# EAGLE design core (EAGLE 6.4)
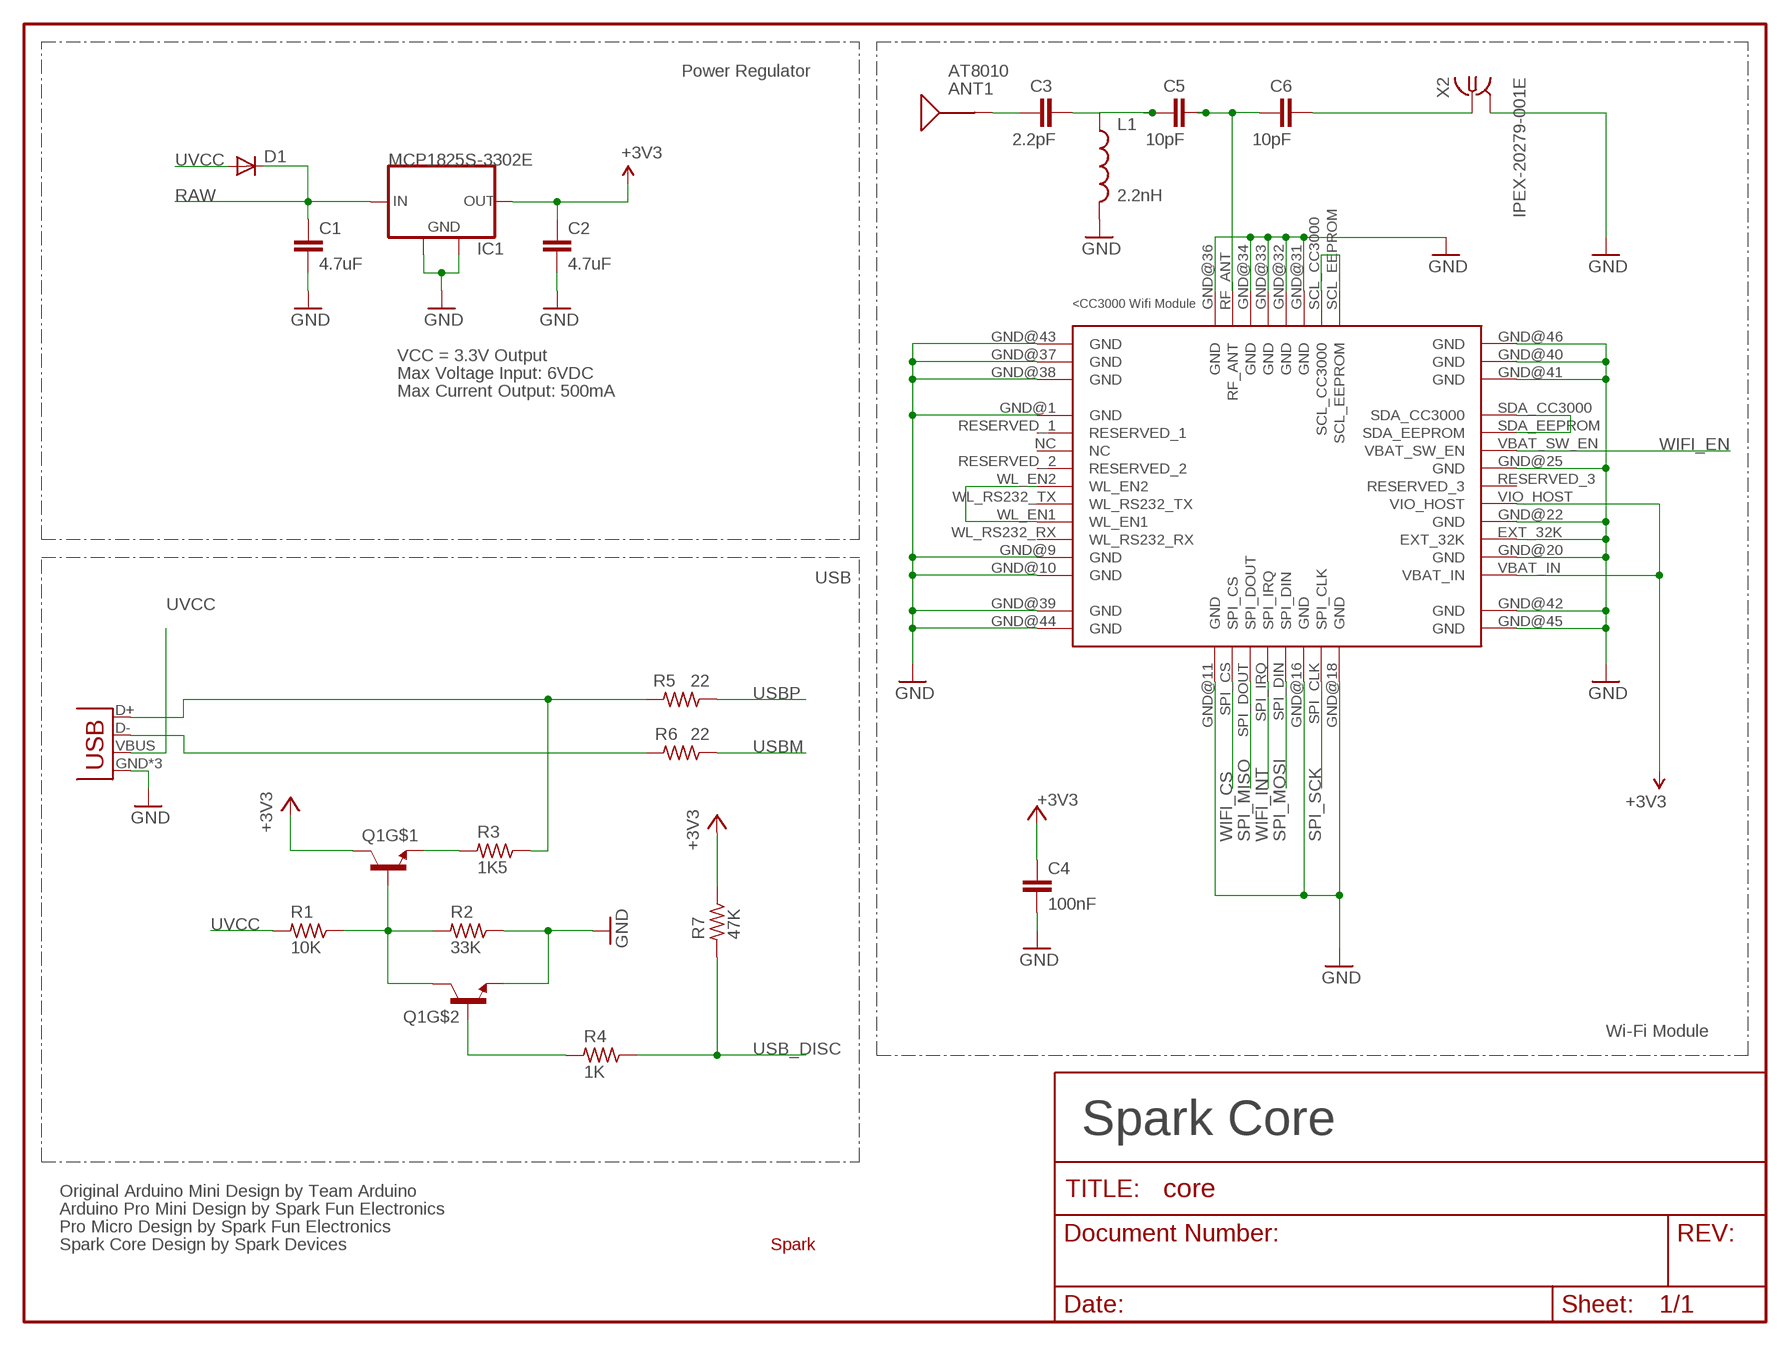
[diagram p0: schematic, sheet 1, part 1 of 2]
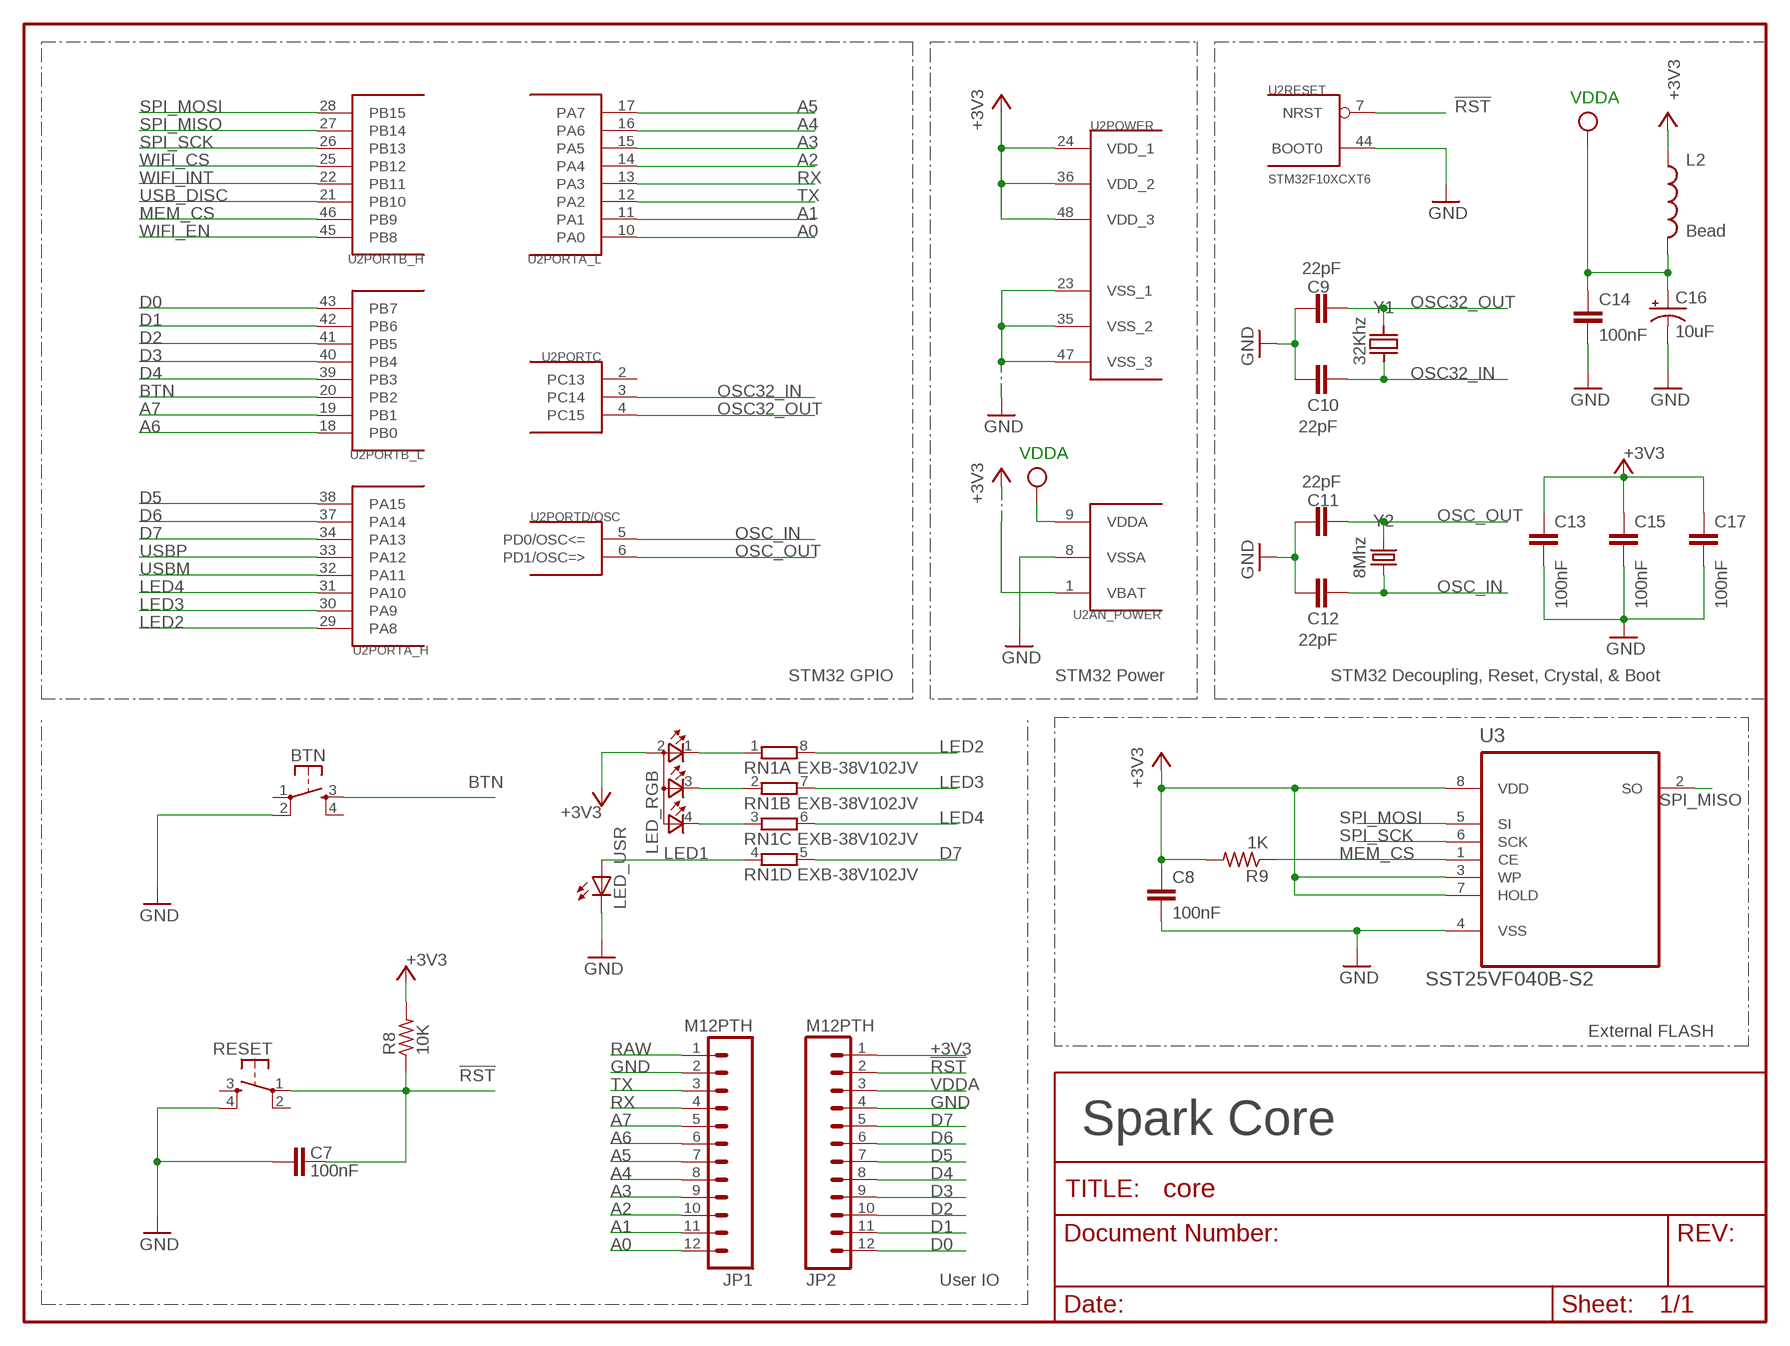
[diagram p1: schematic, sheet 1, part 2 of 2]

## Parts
ANT1  AT8010  [AT8010]
BTN  KMR211GLFS  TAC_SWITCHSMD  [TACTILE_SWITCH_SMD]
C1  4.7uF  C-EUC0603  [C0603]
C2  4.7uF  C-EUC0603  [C0603]
C3  2.2pF  C-EUC0603  [C0603]
C4  100nF  C-EUC0603  [C0603]
C5  10pF  C-EUC0603  [C0603]
C6  10pF  C-EUC0603  [C0603]
C7  100nF  C-EUC0603  [C0603]
C8  100nF  C-EUC0603  [C0603]
C9  22pF  C-EUC0603  [C0603]
C10  22pF  C-EUC0603  [C0603]
C11  22pF  C-EUC0603  [C0603]
C12  22pF  C-EUC0603  [C0603]
C13  100nF  C-EUC0603  [C0603]
C14  100nF  C-EUC0603  [C0603]
C15  100nF  C-EUC0603  [C0603]
C16  10uF  TANT-CAP1206  [EIA3216]
C17  100nF  C-EUC0603  [C0603]
D1  DIODESOD  [SOD-323]
IC1  MCP1825S-3302E  MCP1825S-SOT223  [SOT223]
JP1  M12PTH  [1X12-SMALL-PADS]
JP2  M12PTH  [1X12-SMALL-PADS]
L1  2.2nH  INDUCTOR0603  [0603]
L2  Bead  INDUCTOR0603  [0603]
LED_RGB  TOPLED-3PLCC  [P-LCC-4-3]
LED_USR  LED0603  [LED-0603]
Q1  MMDT3904  [SOT363]
R1  10K  R-US_R0603  [R0603]
R2  33K  R-US_R0603  [R0603]
R3  1K5  R-US_R0603  [R0603]
R4  1K  R-US_R0603  [R0603]
R5  22  R-US_R0603  [R0603]
R6  22  R-US_R0603  [R0603]
R7  47K  R-US_R0603  [R0603]
R8  10K  R-US_R0603  [R0603]
R9  1K  R-US_R0603  [R0603]
RESET  KMR211GLFS  TAC_SWITCHSMD  [TACTILE_SWITCH_SMD]
RN1  EXB-38V102JV  4R-NEXB38V  [EXB38V]
U1  CC3000  [CC3000]
U2  STM32F10XCXT6  [TQFP48]
U3  SST25VF040B-S2  [SOIC127P790X216-8N]
U$1  SPARK_LOGO2  [SPARK_LOGO2]
X1  USB-MICROB  USBUSB-MICROB-SLOT-HOLE  [USB-MICROB-SLOT-HOLE]
X2  IPEX-20279-001E  [IPEX-20279-001E]
Y1  32Khz  Q_FC135  [FC135]
Y2  8Mhz  CRYSTAL5X3  [CRYSTAL-SMD-5X3]

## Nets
!RST: C7.2 JP2.2 R8.1 RESET.1 U2.7(RESET:NRST)
+3V3: C2.1 C4.1 C8.1 C13.1 C15.1 C17.1 IC1.3(OUT) JP2.1 L2.1 LED_RGB.2(A2) Q1.3(C) R7.1 R8.2 R9.2 U1.VBAT_IN U1.VIO_HOST U2.1(AN_POWER:VBAT) U2.24(POWER:VDD_1) U2.36(POWER:VDD_2) U2.48(POWER:VDD_3) U3.3(WP) U3.7(HOLD) U3.8(VDD)
A0: JP1.12 U2.10(PORTA_L:PA0)
A1: JP1.11 U2.11(PORTA_L:PA1)
A2: JP1.10 U2.14(PORTA_L:PA4)
A3: JP1.9 U2.15(PORTA_L:PA5)
A4: JP1.8 U2.16(PORTA_L:PA6)
A5: JP1.7 U2.17(PORTA_L:PA7)
A6: JP1.6 U2.18(PORTB_L:PB0)
A7: JP1.5 U2.19(PORTB_L:PB1)
BTN: BTN.3 U2.20(PORTB_L:PB2)
D0: JP2.12 U2.43(PORTB_L:PB7)
D1: JP2.11 U2.42(PORTB_L:PB6)
D2: JP2.10 U2.41(PORTB_L:PB5)
D3: JP2.9 U2.40(PORTB_L:PB4)
D4: JP2.8 U2.39(PORTB_L:PB3)
D5: JP2.7 U2.38(PORTA_H:PA15)
D6: JP2.6 U2.37(PORTA_H:PA14)
D7: JP2.5 RN1.5 U2.34(PORTA_H:PA13)
GND [vcc]: BTN.2 C1.2 C2.2 C4.2 C7.1 C8.2 C9.2 C10.2 C11.2 C12.2 C13.2 C14.2 C15.2 C16.C(-) C17.2 IC1.2(GND) IC1.4(GND) JP1.2 JP2.4 L1.2 LED_USR.C Q1.1(E) R2.1 RESET.4 U1.EXT_32K U1.GND@1(GND) U1.GND@9(GND) U1.GND@10(GND) U1.GND@11(GND) U1.GND@16(GND) U1.GND@18(GND) U1.GND@20(GND) U1.GND@22(GND) U1.GND@25(GND) U1.GND@31(GND) U1.GND@32(GND) U1.GND@33(GND) U1.GND@34(GND) U1.GND@36(GND) U1.GND@37(GND) U1.GND@38(GND) U1.GND@39(GND) U1.GND@40(GND) U1.GND@41(GND) U1.GND@42(GND) U1.GND@43(GND) U1.GND@44(GND) U1.GND@45(GND) U1.GND@46(GND) U2.8(AN_POWER:VSSA) U2.23(POWER:VSS_1) U2.35(POWER:VSS_2) U2.44(RESET:BOOT0) U2.47(POWER:VSS_3) U3.4(VSS) X1.GND X1.MT1(GND) X1.MT2(GND) X2.2@1(GND) X2.2@2(GND)
LED1: LED_USR.A RN1.4
LED2: RN1.8 U2.29(PORTA_H:PA8)
LED3: RN1.7 U2.30(PORTA_H:PA9)
LED4: RN1.6 U2.31(PORTA_H:PA10)
MEM_CS: R9.1 U2.46(PORTB_H:PB9) U3.1(CE)
N$1: R3.1 R5.2 X1.D+
N$2 [RF]: C6.2 X2.1
N$3 [RF]: ANT1.SIG(SIGNAL) C3.1
N$4 [RF]: C5.2 C6.1 U1.RF_ANT
N$5 [RF]: C3.2 C5.1 L1.1
N$6: R6.2 X1.D-
N$7: U1.SCL_CC3000 U1.SCL_EEPROM
N$8: Q1.2(B) R4.2
N$9: U1.WL_EN1 U1.WL_EN2
N$10: LED_RGB.1(CRED) RN1.1
N$12: LED_RGB.3(CBLUE) RN1.2
N$13: Q1.5(B) Q1.6(C) R1.1 R2.2
N$14: LED_RGB.4(CGREEN) RN1.3
N$15: U1.SDA_CC3000 U1.SDA_EEPROM
N$16: Q1.4(E) R3.2
OSC32_IN: C10.1 U2.3(PORTC:PC14) Y1.X1
OSC32_OUT: C9.1 U2.4(PORTC:PC15) Y1.X2
OSC_IN: C12.1 U2.5(PORTD/OSC:PD0/OSC<=) Y2.1
OSC_OUT: C11.1 U2.6(PORTD/OSC:PD1/OSC=>) Y2.3
RAW [vcc]: C1.1 D1.1(C) IC1.1(IN) JP1.1
RX: JP1.4 U2.13(PORTA_L:PA3)
SPI_MISO: U1.SPI_DOUT U2.27(PORTB_H:PB14) U3.2(SO)
SPI_MOSI: U1.SPI_DIN U2.28(PORTB_H:PB15) U3.5(SI)
SPI_SCK: U1.SPI_CLK U2.26(PORTB_H:PB13) U3.6(SCK)
TX: JP1.3 U2.12(PORTA_L:PA2)
USB_DISC: R4.1 R7.2 U2.21(PORTB_H:PB10)
USBM: R6.1 U2.32(PORTA_H:PA11)
USBP: R5.1 U2.33(PORTA_H:PA12)
UVCC: D1.2(A) R1.2 X1.VBUS
VDDA: C14.1 C16.A(+) JP2.3 L2.2 U2.9(AN_POWER:VDDA) ; supply symbol labelled VCC
WIFI_CS: U1.SPI_CS U2.25(PORTB_H:PB12)
WIFI_EN: U1.VBAT_SW_EN U2.45(PORTB_H:PB8)
WIFI_INT: U1.SPI_IRQ U2.22(PORTB_H:PB11)
Unconnected: BTN.1 BTN.4 RESET.2 RESET.3 U1.NC U1.RESERVED_1 U1.RESERVED_2 U1.RESERVED_3 U1.WL_RS232_RX U1.WL_RS232_TX U2.2(PORTC:PC13)

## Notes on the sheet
- Power Regulator
- VDDA
- VCC = 3.3V Output
- Max Voltage Input: 6VDC
- Max Current Output: 500mA
- VDDA
- USB
- STM32 GPIO | STM32 Power | STM32 Decoupling, Reset, Crystal, & Boot
- Wi-Fi Module | External FLASH
- Spark Core | Spark Core
- Original Arduino Mini Design by Team Arduino
- Arduino Pro Mini Design by Spark Fun Electronics
- Pro Micro Design by Spark Fun Electronics
- Spark Core Design by Spark Devices
- User IO

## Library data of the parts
ANT1 = Spark:AT8010: AT8010 Series Multilayer Chip Antenna
BTN RESET = Spark:TAC_SWITCH: SMD Tactiile Switch
C1-C15 C17 = rcl:C-EU: CAPACITOR, European symbol
C16 = Spark:TANT-CAP: Tantalum SMT
D1 = SparkFun:DIODE: Diode
IC1 = Spark:MCP1825S: 500 mA, Low Voltage, Low Quiescent Current LDO Regulator
JP1 JP2 = Spark:M12: Header 12 Standard 12-pin 0.1" header. Use with straight break away headers (SKU : PRT-00116), right angle break away headers (PRT-00553), swiss pins (PRT-00743), machine pins (PRT-00117), and female headers (PRT-00115).
L1 L2 = SparkFun-Passives:INDUCTOR: Inductors
LED_RGB = Spark:TOPLED-3: Cree CLVBA-FKA
LED_USR = SparkFun:LED: LEDs
Q1 = SparkFun-DiscreteSemi:MMDT3904: Dual NPN transistor
R1-R9 = rcl:R-US_: RESISTOR, American symbol
RN1 = resistor-dil:4R-N: Array Chip Resistor Source: RS Component / Phycomp; OC_FARNELL: unknown; OC_NEWARK: unknown
U1 = CC3000:CC3000
U2 = stm32:STM32F10XCXT6: ST STM32F101/103 48pin LQFP
U3 = Spark:SST25VF040B: 4 Mbit SPI Serial Flash
U$1 = Spark:SPARK_LOGO2
X1 = Spark:USB
X2 = Spark:IPEX-20279-001E: Ultra Miniature Coaxial SMT RF Receptacle
Y1 = Spark:Q
Y2 = SparkFun-FreqCtrl:CRYSTAL: Various standard crystals. Proven footprints. Spark Fun Electronics SKU : COM-00534

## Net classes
2 RF: width 0.635 mm, clearance 0.762 mm

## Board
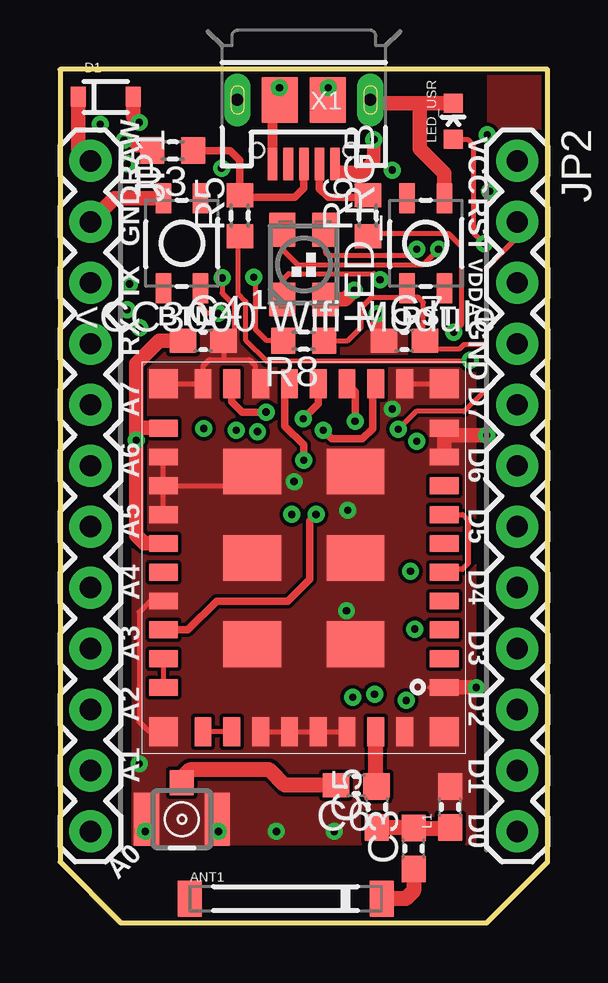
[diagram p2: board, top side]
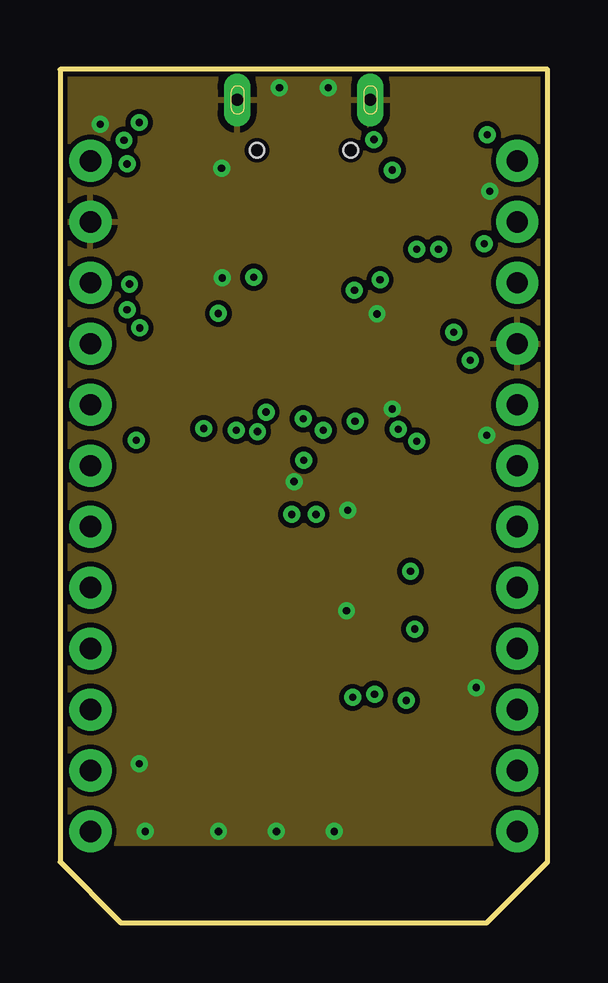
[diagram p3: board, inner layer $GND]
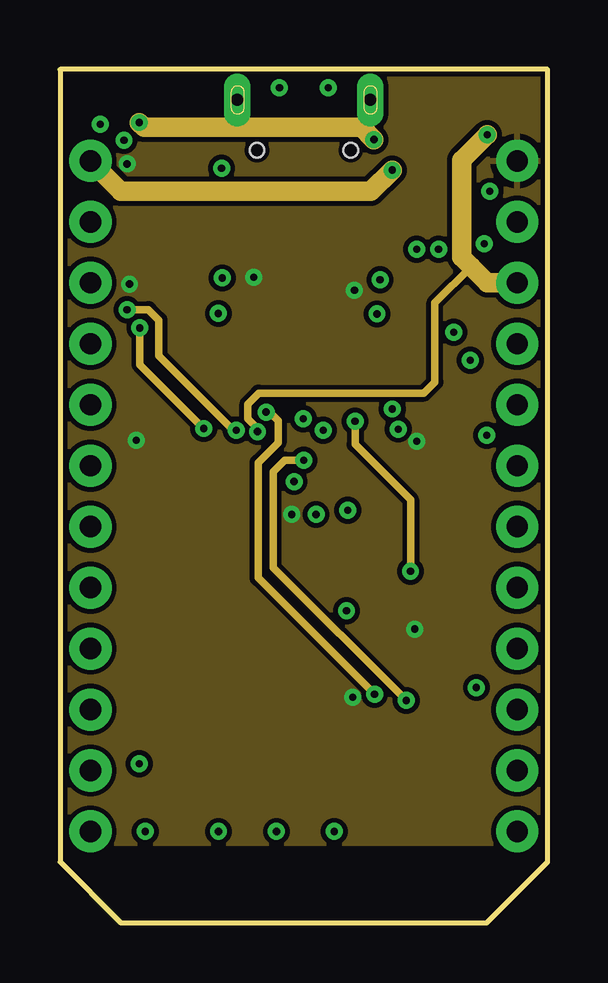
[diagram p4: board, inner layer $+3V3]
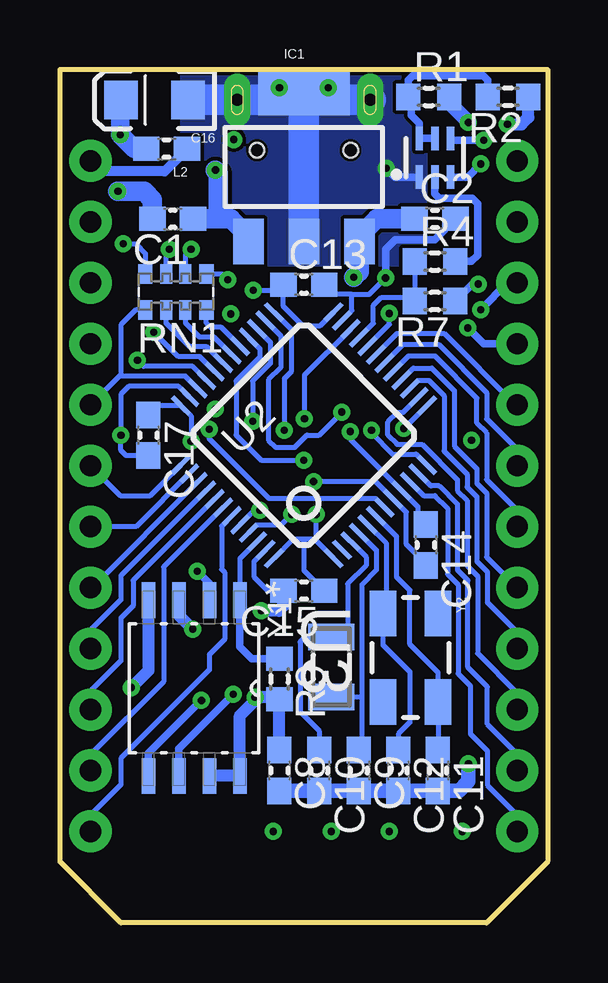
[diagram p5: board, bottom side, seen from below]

Size 20.32 x 35.56 mm. Coordinates in mm from the lower left corner, seen from the top.
Outline: 0,35.56 0,2.54 2.54,0 17.78,0 20.32,2.54 20.32,35.56 0,35.56
Copper layers (1+2*15+16): Top 0.035mm / dielectric 1.5mm / $GND 0.035mm / dielectric 0.15mm / $+3V3 0.035mm / dielectric 0.2mm / Bottom 0.035mm
Design rules "spark": minimum track width 6mil, minimum drill 0.3mm, track to track 6mil, track to pad 6mil, pad to pad 6mil, via to via 6mil, smd to smd 6mil, copper to edge 6mil, drill to drill 6mil, minimum pad ring 12mil, minimum via ring 8mil, stop-mask expansion 4mil, vias tented up to drill 20mil, thermal gap 10mil

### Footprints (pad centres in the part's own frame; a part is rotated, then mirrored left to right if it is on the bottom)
AT8010 = smd 1 x 1.5: NC -4,0; SIG 4,0
TACTILE_SWITCH_SMD = smd 1.25 x 0.65: 1 -1.875,0.775; 2 1.875,0.775; 3 -1.875,-0.775; 4 1.875,-0.775
C0603 = smd 1.1 x 1: 1 -0.85,0; 2 0.85,0
EIA3216 = smd 1.4 x 1.6: A 1.4,0; C -1.4,0
SOD-323 = smd 0.63 x 0.83: 1 -1.15,0; 2 1.15,0
SOT223 = smd 1.27 x 1.905: 1 -2.311,-3.099; 2 0,-3.099; 3 2.311,-3.099 | smd 3.81 x 1.905: 4 0,3.099
1X12-SMALL-PADS = drill 0.889 pad 1.753: 1 0,0; 2 2.54,0; 3 5.08,0; 4 7.62,0; 5 10.16,0; 6 12.7,0; 7 15.24,0; 8 17.78,0; 9 20.32,0; 10 22.86,0; 11 25.4,0; 12 27.94,0
0603 = smd 1.1 x 1: 1 -0.85,0; 2 0.85,0
P-LCC-4-3 = smd 1.1 x 1.4: 1 -0.9,-1.45; 2 0.9,-1.45; 3 0.9,1.45; 4 -0.9,1.45
LED-0603 = smd 0.8 x 0.8: A 0,-0.75; C 0,0.75
SOT363 = smd 0.3 x 0.99: 1 -0.65,-0.8; 2 0,-0.8; 3 0.65,-0.8; 4 0.65,0.81; 5 0,0.81; 6 -0.65,0.81
R0603 = smd 1 x 1.1: 1 -0.85,0; 2 0.85,0
EXB38V = smd 0.6 x 0.8: 1 -1.275,-0.75; 4 1.275,-0.75; 5 1.275,0.75; 8 -1.275,0.75 | smd 0.5 x 0.8: 2 -0.4,-0.75; 3 0.4,-0.75; 6 0.4,0.75; 7 -0.4,0.75
CC3000 = smd 1.2 x 0.7: EXT_32K 5.85,-2.97; GND@1 -5.85,5.43; GND@9 -5.85,-4.17; GND@10 -5.85,-5.37; GND@20 5.85,-4.17; GND@22 5.85,-1.77; GND@25 5.85,1.83; NC -5.85,3.03; RESERVED_1 -5.85,4.23; RESERVED_2 -5.85,1.83; RESERVED_3 5.85,0.63; SDA_CC3000 5.85,5.43; SDA_EEPROM 5.85,4.23; VBAT_IN 5.85,-5.37; VBAT_SW_EN 5.85,3.03; VIO_HOST 5.85,-0.57; WL_EN1 -5.85,-1.77; WL_EN2 -5.85,0.63; WL_RS232_RX -5.85,-2.97; WL_RS232_TX -5.85,-0.57 | smd 0.7 x 1.2: GND@11 -4.2,-7.22; GND@16 1.8,-7.22; GND@18 4.2,-7.22; GND@31 1.8,7.28; GND@32 0.6,7.28; GND@33 -0.6,7.28; GND@34 -1.8,7.28; GND@36 -4.2,7.28; RF_ANT -3,7.28; SCL_CC3000 3,7.28; SCL_EEPROM 4.2,7.28; SPI_CLK 3,-7.22; SPI_CS -3,-7.22; SPI_DIN 0.6,-7.22; SPI_DOUT -1.8,-7.22; SPI_IRQ -0.6,-7.22 | smd 2.4 x 1.9: GND@37 -2.15,3.63; GND@38 -2.15,0.03; GND@39 -2.15,-3.57; GND@40 2.15,3.63; GND@41 2.15,0.03; GND@42 2.15,-3.57 | smd 1.2 x 1.2: GND@43 -5.85,7.28; GND@44 -5.85,-7.22; GND@45 5.85,-7.22; GND@46 5.85,7.28
TQFP48 = smd 0.2 x 1: 1 -2.75,-4.5; 2 -2.25,-4.5; 3 -1.75,-4.5; 4 -1.25,-4.5; 5 -0.75,-4.5; 6 -0.25,-4.5; 7 0.25,-4.5; 8 0.75,-4.5; 9 1.25,-4.5; 10 1.75,-4.5; 11 2.25,-4.5; 12 2.75,-4.5; 25 2.75,4.5; 26 2.25,4.5; 27 1.75,4.5; 28 1.25,4.5; 29 0.75,4.5; 30 0.25,4.5; 31 -0.25,4.5; 32 -0.75,4.5; 33 -1.25,4.5; 34 -1.75,4.5; 35 -2.25,4.5; 36 -2.75,4.5 | smd 1 x 0.2: 13 4.5,-2.75; 14 4.5,-2.25; 15 4.5,-1.75; 16 4.5,-1.25; 17 4.5,-0.75; 18 4.5,-0.25; 19 4.5,0.25; 20 4.5,0.75; 21 4.5,1.25; 22 4.5,1.75; 23 4.5,2.25; 24 4.5,2.75; 37 -4.5,2.75; 38 -4.5,2.25; 39 -4.5,1.75; 40 -4.5,1.25; 41 -4.5,0.75; 42 -4.5,0.25; 43 -4.5,-0.25; 44 -4.5,-0.75; 45 -4.5,-1.25; 46 -4.5,-1.75; 47 -4.5,-2.25; 48 -4.5,-2.75
SOIC127P790X216-8N = smd 1.499 x 0.559: 1 -3.658,1.905; 2 -3.658,0.635; 3 -3.658,-0.635; 4 -3.658,-1.905; 5 3.658,-1.905; 6 3.658,-0.635; 7 3.658,0.635; 8 3.658,1.905
USB-MICROB-SLOT-HOLE = smd 0.4 x 1.35: D+ 0,2.675; D- -0.65,2.675; GND 1.3,2.675; ID 0.65,2.675; VBUS -1.3,2.675 | drill 0.5 pad 1.1 long: MT1 -2.775,0; MT2 2.775,0 | smd 1.5 x 1.9: P$1 -1,0; P$2 1,0.01 | hole 0.6: -1.95,2.1; 1.95,2.1
IPEX-20279-001E = smd 1 x 1.05: 1 0,1.528 | smd 1.05 x 2.2: 2@1 -1.475,0; 2@2 1.475,0
FC135 = smd 1.1 x 1.9: X1 -1.25,0; X2 1.25,0
CRYSTAL-SMD-5X3 = smd 1.9 x 1.1: 1 -1.85,-1.15; 2 1.85,-1.15; 3 1.85,1.15; 4 -1.85,1.15

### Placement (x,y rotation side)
ANT1  9.4,1.02 0 top
BTN  5.08,28.32 90 top
C1  15.62,29.34 180 bottom
C2  4.7,29.34 0 bottom
C3  14.73,3.1 90 top
C4  5.97,24.26 0 top
C5  13.21,4.83 90 top
C6  12.34,5.74 180 top
C7  14.35,24.26 0 top
C8  11.18,6.35 270 bottom
C9  7.87,6.35 270 bottom
C10  9.53,6.35 270 bottom
C11  4.57,6.35 270 bottom
C12  6.22,6.35 270 bottom
C13  10.16,26.59 0 bottom
C14  5.08,15.75 270 bottom
C15  10.16,13.84 180 bottom
C16  16.38,34.29 180 bottom
C17  16.64,20.32 270 bottom
D1  1.91,34.42 0 top
IC1  10.16,31.5 0 bottom
JP1  1.27,31.75 270 top
JP2  19.05,31.75 270 top
L1  16.26,4.83 90 top
L2  15.88,32.26 180 bottom
LED_RGB  10.16,27.43 0 top
LED_USR  16.38,33.4 0 top
Q1  4.7,31.88 0 bottom
R1  4.95,34.42 0 bottom
R2  1.65,34.42 180 bottom
R3  4.7,32.18 180 top
R4  4.7,27.56 0 bottom
R5  7.49,29.46 90 top
R6  12.83,29.46 90 top
R7  4.7,25.91 180 bottom
R8  10.16,24.26 180 top
R9  11.18,10.16 270 bottom
RESET  15.24,28.32 90 top
RN1  15.49,26.29 180 bottom
U1  10.16,15.24 180 top
U2  10.16,20.32 45 bottom
U3  14.73,9.78 270 bottom
U$1  17.78,33.02 0 top
X1  10.16,34.29 180 top
X2  5.08,4.32 0 top
Y1  9.02,10.67 270 bottom
Y2  5.71,11.05 270 bottom

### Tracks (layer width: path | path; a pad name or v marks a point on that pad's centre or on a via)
!RST  (via drill 0.3)
  Top 0.203: 17.75,24.08 17.75,27.28 19.05,28.57 JP2.2 | 17.75,24.08 17.75,22.22 16.84,21.31 14.83,21.31 v14.1,20.57 | 17.75,24.08 17.73,24.11 16.84,24.11 16.66,23.93 15.53,23.93 C7.2 15.14,24.32 15.14,25.86 14.94,26.06 14.46,26.06 | R8.1 11.99,24.26 12.55,24.82 12.55,25.63 12.98,26.06 14.46,26.06 | 14.46,26.06 RESET.1
  Bottom 0.203: U2.7 7.17,17.68 11.61,17.68 14.1,20.17 v14.1,20.57
+3V3  (via drill 0.3)
  Top 0.203: R8.2 8.61,24.26 8.15,24.71 8.15,26.82 v8.08,26.9
  Top 0.61: U1.VIO_HOST 3.52,15.81 3.17,16.15 v3.17,20.12 3.17,20.62 | 3.17,20.62 3.17,23.29 4.14,24.26 C4.1 | U1.VBAT_IN 4.29,20.62 3.17,20.62 | LED_RGB.2 11.88,25.98 v12.27,26.36
  Bottom 0.203: U2.1 9.71,15.98 | 9.71,15.98 10.16,15.98 | 10.16,15.98 10.62,15.98 U2.48 | 10.16,15.98 10.16,14.69 C15.1 | U2.24 9.5,24.87 10.19,24.87 11.01,25.69 C13.1 11.24,26.36 v12.27,26.36 | C17.1 16.25,21.56 U2.36 14.86,21.13 v14.86,20.07 | 9.71,15.98 9.65,16.03 v9.65,17.02
  Bottom 0.305: R7.1 3.14,26.62 v2.9,26.62 | Q1.3 3.34,31.08 v2.79,31.62
  Bottom 0.406: L2.1 15.96,31.32 18.62,31.32 JP2.1
  Bottom 0.508: U3.7 U3.8 12.83,8.64 12.19,9.27 v12.19,9.4 11.6,9.4 11.34,9.14 R9.2 C8.1 | v14.78,12.24 15.37,12.83 U3.3
  Bottom 0.813: C2.1 7.11,29.34 7.85,28.6 IC1.3 7.85,27.13 v8.08,26.9
  pour $+3V3 (isolate 0.203): 0,35.56 20.32,35.56 20.32,3.3 0,3.3
A0
  Bottom 0.203: U2.10 5.17,17.8 4.7,17.8 4.17,17.27 4.17,14.53 3.73,14.1 3.73,10.39 3.23,9.88 3.23,7.87 2.52,7.16 2.52,5.74 1.27,4.5 JP1.12
A1
  Bottom 0.203: U2.11 4.87,18.21 4.52,18.21 3.76,17.45 3.76,14.71 3.33,14.27 3.33,10.64 2.52,9.83 2.52,8.28 1.27,7.04 JP1.11
A2
  Bottom 0.203: U2.14 6.04,21.26 6.27,21.26 6.66,20.88 6.66,20.32 6.27,19.94 5.23,19.94 3.76,18.47 3.76,18.01 3.35,17.6 3.35,14.88 2.92,14.45 2.92,11.23 1.27,9.58 JP1.10
A3
  Bottom 0.203: U2.15 5.4,22.61 4.95,22.61 4.32,21.97 4.32,19.66 3.35,18.69 3.35,18.16 2.95,17.75 2.95,15.06 2.52,14.63 2.52,13.36 1.27,12.12 JP1.9
A4
  Bottom 0.203: U2.16 5.6,23.11 4.83,23.11 3.89,22.17 3.89,19.86 2.95,18.92 2.95,18.31 2.54,17.91 2.54,15.24 JP1.8
A5
  Bottom 0.203: U2.17 5.8,23.62 4.7,23.62 2.95,21.87 2.95,20.83 2.54,20.42 2.54,18.47 1.27,17.2 JP1.7
A6
  Bottom 0.203: U2.18 6.02,24.11 4.55,24.11 2.54,22.1 2.54,21.01 1.27,19.74 JP1.6
A7
  Bottom 0.203: U2.19 6.27,24.56 4.32,24.56 1.35,21.59 JP1.5
BTN  (via drill 0.3)
  Top 0.203: 5.84,26.43 BTN.3 5.87,26.43 5.87,25.65 6.13,25.39 v6.6,25.39
  Bottom 0.203: U2.20 6.6,24.94 v6.6,25.39
D0
  Bottom 0.203: JP2.12 19.05,4.5 17.78,5.77 17.78,6.86 14.1,10.54 14.1,11.18 13.46,11.81 13.46,14.61 13.59,14.73 13.59,16.54 U2.43
D1
  Bottom 0.203: U2.42 16,14.83 16,10.06 19.05,7.01 JP2.11
D2
  Bottom 0.203: U2.41 17.27,14.27 17.27,13.21 17.78,12.7 17.78,10.92 19.05,9.65 JP2.10
D3
  Bottom 0.203: U2.40 17.77,14.48 17.78,14.48 17.78,13.46 19.05,12.19 JP2.9
D4
  Bottom 0.203: U2.39 18.98,13.97 JP2.8
D5
  Bottom 0.203: U2.38 17.15,16.51 JP2.7
D6
  Bottom 0.203: U2.37 16.59,17.78 17.78,17.78 JP2.6
D7
  Bottom 0.203: U2.34 15.1,22.78 17.86,22.78 | RN1.5 17.16,25.54 17.78,24.92 17.78,22.86 17.86,22.78 | 17.86,22.78 JP2.5
GND  (via drill 0.3)
  Top 0.203: U1.GND@43 16.01,8.12 | U1.GND@1 15.4,9.81 | U1.GND@34 U1.GND@33 U1.GND@32 U1.GND@31 8.36,8.4 | U1.GND@22 U1.EXT_32K | U1.GND@45 U1.GND@18 | U1.GND@38 12.41,15.11 | U1.GND@25 4.49,13.59 3.94,13.59 3.3,12.95 3.3,8.38 3.68,8 4.27,8 U1.GND@46 | U1.GND@11 U1.GND@44 | U1.EXT_32K U1.GND@20 | U1.EXT_32K 7.41,18.21 U1.GND@42 | U1.GND@18 | 8.26,21.97 8.26,22.36 U1.GND@16 8.13,22.69 8.13,23.24 7.9,23.47 6.83,23.47 | U1.GND@18 5.96,23.21 6.22,23.47 6.83,23.47 | 6.83,23.47 6.82,23.48 C4.2 7.26,24.7 7.26,25.73 6.76,26.24 v6.76,26.87 | 12.06,17.27 12.06,17.4
  Top 0.406: X1.GND 8.86,34.51 v9.14,34.8
  Top 0.508: v13.21,25.38 13.21,24.55 C7.1
  Top 0.61: U1.GND@1 v17.34,9.81 v17.35,9.8 | U1.GND@9 U1.GND@10 16.3,20.32 v17.78,20.32 | RESET.4 16.02,31.23 14.99,32.26 14.99,34.15 | LED_USR.C 14.99,34.15 | 14.99,34.15 13.07,34.15 X1.MT1 | BTN.2 2.26,30.2 JP1.2
  Bottom 0.203: U2.35 15.37,22.35 17.45,22.35 17.78,22.02 v17.78,20.32 17.78,19.68 17.57,19.47 C17.2 | U2.47 12.24,15.05 12.24,14.43 11.66,13.84 C15.2 | 8.15,26.19 7.44,26.19 v6.76,26.87 | U2.23 8.15,25.51 8.15,26.19 | C14.2 5.08,14.96 5.89,15.77 5.89,17.11 U2.8 7.17,18.39 v9.75,18.39 | 8.15,26.19 8.9,26.19 C13.2 | U2.44 12.22,17.2 v11.99,17.2
  Bottom 0.305: 10.16,34.67 IC1.4 | Q1.1 6.36,31.08 v6.73,31.45 | C2.2 4.71,28.47 6.35,28.47 6.76,28.07 v6.76,26.87
  Bottom 0.508: U3.4 16.64,10.52 v17.35,9.8 | v11.94,13 11.2,13 11.01,13.2 C15.2 | v1.68,33.27 1.09,33.27 0.8,33.56 R2.1 0.81,34.41
  Bottom 0.61: C8.2 C10.2 C9.2 C12.2 C11.2 3.69,5.5 3.3,5.89 v3.3,6.63
  Bottom 0.813: C1.2 16.47,30.14 16.82,30.48 v17.91,30.48 | 10.16,34.8 IC1.4
  Bottom 1.27: IC1.2 IC1.4 | 7.37,34.29 X1.MT1 C16.C
  other vias: 3.56,3.81 6.6,3.81 9.02,3.81 11.43,3.81 13.84,21.41 11.18,34.8
  pour $GND (isolate 0.203): 0,35.56 20.32,35.56 20.32,3.3 0,3.3
  pour Top (no thermals): 3.05,3.3 3.05,24.64 17.27,24.64 17.27,3.3
  pour Bottom (no thermals): 5.08,35.56 15.24,35.56 15.24,27.43 5.08,27.43
LED1  (via drill 0.3)
  Top 0.203: LED_USR.A 16.98,32.65 17.22,32.41 17.22,28.75 v17.68,28.3
  Bottom 0.203: v17.68,28.3 17.17,28.3 16.76,27.89 RN1.4
LED2
  Bottom 0.203: U2.29 13.6,24.82 14.05,24.82 14.22,24.99 RN1.8
LED3
  Bottom 0.203: U2.30 13.9,24.41 14.5,24.41 15.09,24.99 RN1.7
LED4
  Bottom 0.203: U2.31 14.2,24 14.91,24 15.9,24.99 RN1.6
MEM_CS
  Bottom 0.203: U2.46 12.83,15.18 U3.1
  Bottom 0.305: U3.1 12.83,11.51 12.33,11.01 R9.1
N$1
  Top 0.305: R3.1 7.09,32.18 7.49,31.77 R5.2 7.58,30.23 9.78,30.23 10.16,30.61 X1.D+
N$2
  Top 0.635: C6.2 9.37,5.74 8.74,6.38 5.4,6.38 5.08,6.06 X2.1
N$3
  Top 0.635: C3.1 14.73,1.33 14.41,1.02 ANT1.SIG
N$4
  Top 0.406: 13.21,5.74 C6.1
  Top 0.635: C6.1 13.16,5.78 U1.RF_ANT | 13.21,5.74 C5.2
N$5
  Top 0.635: C5.1 14.71,3.98 C3.2 16.23,3.95 L1.1
N$6
  Top 0.305: R6.2 12.74,30.23 11.18,30.23 10.81,30.59 X1.D-
N$7
  Top 0.203: U1.SCL_CC3000 U1.SCL_EEPROM
N$8
  Bottom 0.305: Q1.2 4.7,30.38 4.52,30.2 3.15,30.2 2.92,29.97 2.92,27.81 3.17,27.56 R4.2
N$9
  Top 0.203: U1.WL_EN1 16.77,17.01 17.02,16.76 17.02,14.99 16.76,14.73 16.13,14.73 U1.WL_EN2
N$10  (via drill 0.3)
  Top 0.203: LED_RGB.1 9.26,26.79 9.53,27.05 13.08,27.05 v13.34,26.8
  Bottom 0.203: RN1.1 13.58,27.04 v13.34,26.8
N$11
  pour Top: 17.91,35.56 20.32,35.56 20.32,33.15 17.91,33.15
N$12  (via drill 0.3)
  Top 0.203: LED_RGB.3 11.06,27.93 11.18,27.81 14.61,27.81 v14.86,28.07
  Bottom 0.203: v14.86,28.07 15.09,27.83 RN1.2
N$13
  Bottom 0.305: Q1.5 Q1.6 5.35,33.31 5.69,33.66 5.69,34.3 R1.1 5.8,35.12 5.61,35.31 2.69,35.31 2.5,35.12 R2.2
N$14  (via drill 0.3)
  Top 0.203: LED_RGB.4 9.26,28.08 9.91,27.43 15.14,27.43 v15.77,28.07
  Bottom 0.203: RN1.3 15.89,27.95 v15.77,28.07
N$15
  Top 0.203: U1.SDA_EEPROM U1.SDA_CC3000
N$16  (via drill 0.3)
  Top 0.305: 3.76,32.18 R3.2 3.77,32.26 3.2,32.26 2.85,32.61 v2.67,32.61
  Bottom 0.305: Q1.4 3.98,32.61 v2.67,32.61
OSC32_IN
  Bottom 0.203: U2.3 7.57,15.25 7.57,14.88 8.33,14.12 8.33,12.27 8.43,12.17 8.77,12.17 Y1.X1 10.1,11.92 10.31,11.71 10.31,8.79 9.53,8 C10.1
OSC32_OUT
  Bottom 0.203: U2.4 7.14,15.53 7.14,14.71 7.75,14.1 7.75,9.42 | 7.75,9.42 7.75,7.33 C9.1 | Y1.X2 7.75,9.42
OSC_IN
  Bottom 0.203: U2.5 6.73,15.83 6.73,13.03 Y2.1 6.87,11.59 5.74,10.46 5.74,8.36 6.22,7.87 C12.1
OSC_OUT
  Bottom 0.203: U2.6 6.3,16.11 6.3,14.43 5.74,13.87 5.74,11.61 4.57,10.43 Y2.3 | 4.57,9.21 Y2.3 | Y2.3 C11.1
RAW  (via drill 0.3)
  Top 0.61: D1.1 0.76,32.27 JP1.1
  $+3V3 0.813: v13.84,31.37 12.95,30.48 2.54,30.48 JP1.1
  Bottom 0.813: IC1.1 12.47,28.6 13.21,29.34 13.72,29.34 | 13.72,29.34 C1.1 | v13.84,31.37 13.72,31.24 13.72,29.34
RX  (via drill 0.3)
  $+3V3 0.305: v3.33,24.79 3.33,23.26 v5.99,20.6
  Bottom 0.203: U2.13 v5.99,20.6
  Bottom 0.305: v3.33,24.79 2.67,24.13 JP1.4
SPI_MISO  (via drill 0.3)
  Top 0.305: U1.SPI_DOUT 12.29,22.13 v12.29,20.9
  $+3V3 0.305: v12.29,20.9 12.29,19.94 14.61,17.63 v14.61,14.66
  Bottom 0.203: U2.27 11.56,24.19 11.56,23.32 12.29,22.58 v12.29,20.9
  Bottom 0.305: U3.2 14.1,14.15 v14.61,14.66
SPI_MOSI  (via drill 0.3)
  Top 0.305: U1.SPI_DIN 9.37,22.27 9.37,20.7 10.16,19.91 v10.16,19.28
  $+3V3 0.305: v14.43,9.27 8.89,14.81 8.89,18.8 9.37,19.28 v10.16,19.28
  Bottom 0.203: U2.28 11.99,23.92 11.99,23.57 12.98,22.58 12.98,20.32 11.94,19.28 v10.16,19.28
  Bottom 0.305: U3.5 16.64,7.06 v14.43,9.27
SPI_SCK  (via drill 0.3)
  Top 0.305: U1.SPI_CLK 7.16,21.72 7.59,21.29 v8.59,21.29
  $+3V3 0.305: v13.11,9.53 8.26,14.38 8.26,19.18 9.09,20.02 9.09,20.93 8.74,21.29 v8.59,21.29
  Bottom 0.203: 8.59,21.21 v8.59,21.29 8.59,21.26 9.53,20.32 10.03,20.32 10.54,19.81 11.33,19.81 11.63,20.12 11.63,22.63 11.12,23.14 11.12,24.47 U2.26
  Bottom 0.305: U3.6 15.37,7.26 v13.11,9.53
TX  (via drill 0.3)
  $+3V3 0.305: v2.79,25.55 3.68,25.55 4.12,25.12 4.12,23.62 7.21,20.52 v7.34,20.52
  Bottom 0.203: U2.12 5.48,19.53 6.48,19.53 7.34,20.4 v7.34,20.52
  Bottom 0.305: v2.79,25.55 1.68,26.67 JP1.3
USB_DISC
  Bottom 0.203: U2.21 7.26,24.98 7.26,25.73 6.93,26.06 5.7,26.06 R7.2 R4.1
USBM  (via drill 0.3)
  Top 0.203: R6.1 12.94,28.73 16.18,28.73 16.71,28.19 16.71,24.92 v16.41,24.61
  Bottom 0.203: U2.32 14.5,23.6 15.39,23.6 v16.41,24.61
USBP  (via drill 0.3)
  Top 0.203: v17.09,23.44 17.04,23.39 8.61,23.39 7.75,24.26 7.75,25.88 7.42,26.21 7.42,28.54 R5.1
  Bottom 0.203: U2.33 14.8,23.19 16.84,23.19 v17.09,23.44
UVCC  (via drill 0.3)
  Top 0.305: 11.46,31.52 X1.VBUS
  Top 0.406: 11.73,31.27 11.71,31.27 11.46,31.52
  Top 0.559: 11.73,31.27 12.6,31.27 13.08,31.75 v13.08,32.64
  Top 0.61: D1.2 3.06,33.6 v3.3,33.35
  $+3V3 0.813: v13.08,32.64 12.57,33.15 3.5,33.15 v3.3,33.35
  Bottom 0.61: v3.3,33.35 3.3,33.38 4.1,34.18 R1.2
VDDA  (via drill 0.3)
  $+3V3 0.305: 17.13,27.34 15.62,25.83 15.62,22.53 15.16,22.07 8.28,22.07 7.82,21.61 7.82,21.01 8.23,20.6 v8.23,20.47
  $+3V3 0.813: v17.8,32.84 16.74,31.77 16.74,27.74 17.13,27.34 17.8,26.67 JP2.3
  Bottom 0.203: C14.1 5.41,16.93 5.41,17.34 U2.9 8.23,20.16 v8.23,20.47
  Bottom 0.762: C16.A 17.8,34.27 v17.8,32.84 17.22,32.26 L2.2
WIFI_CS  (via drill 0.3)
  Top 0.203: U1.SPI_CS 12.91,22.7
  Top 0.305: v10.97,20.52 11.33,20.17 12.6,20.17 13.03,20.6 13.03,22.33 U1.SPI_CS
  Bottom 0.203: U2.25 10.69,24.74 10.69,22.96 10.97,22.68 v10.97,20.52
WIFI_EN  (via drill 0.3)
  Top 0.203: 4.33,12.19 U1.VBAT_SW_EN
  Top 0.305: U1.VBAT_SW_EN 5.33,12.21 6.53,13.41 9.5,13.41 10.41,14.33 10.41,16.76 v10.67,17.02
  Bottom 0.203: U2.45 12.13,16.59 11.1,16.59 v10.67,17.02
WIFI_INT  (via drill 0.3)
  Top 0.305: v10.13,21.01 10.76,21.63 U1.SPI_IRQ
  Bottom 0.203: U2.22 10.13,22.82 v10.13,21.01

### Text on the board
tPlace: VCC | RAW | RST | GND | VDDA | TX | GND | BTN | RST | RX | D7 | A7 | D6 | A6 | D5 | A5 | D4 | A4 | D3 | A3 | D2 | A2 | D1 | A1 | D0 | A0

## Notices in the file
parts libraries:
SparkFun-Passives: Licensing: CC v3.0 Share-Alike You are welcome to use this library for commercial purposes.
